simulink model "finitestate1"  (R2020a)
settings: Solver=FixedStepDiscrete  StartTime=0.0  StopTime=30  FixedStep=1  RelTol=1e-3  EnableMultiTasking=on

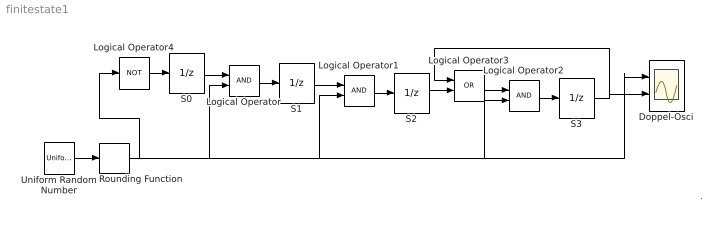
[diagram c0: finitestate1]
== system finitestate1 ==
  note: .
  Doppel-Osci : Scope  NumInputPorts=2
  Logical Operator : Logic
  Logical Operator1 : Logic
  Logical Operator2 : Logic
  Logical Operator3 : Logic  Operator=OR
  Logical Operator4 : Logic  Operator=NOT
  Rounding Function : Rounding  Operator=round
  S0 : UnitDelay  InitialCondition=1  SampleTime=-1  HasFrameUpgradeWarning=on
  S1 : UnitDelay  SampleTime=-1  HasFrameUpgradeWarning=on
  S2 : UnitDelay  SampleTime=-1  HasFrameUpgradeWarning=on
  S3 : UnitDelay  SampleTime=-1  HasFrameUpgradeWarning=on
  Uniform Random Number : UniformRandomNumber  Minimum=0  SampleTime=0
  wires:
  Uniform Random Number/1 -> Rounding Function/1
  S0/1 -> Logical Operator/1
  Rounding Function/1 -> Logical Operator/2, Logical Operator1/2, Logical Operator2/2, Doppel-Osci/1, Logical Operator4/1
  Logical Operator/1 -> S1/1
  S1/1 -> Logical Operator1/1
  Logical Operator1/1 -> S2/1
  Logical Operator2/1 -> S3/1
  S3/1 -> Logical Operator3/1, Doppel-Osci/2
  S2/1 -> Logical Operator3/2
  Logical Operator3/1 -> Logical Operator2/1
  Logical Operator4/1 -> S0/1
